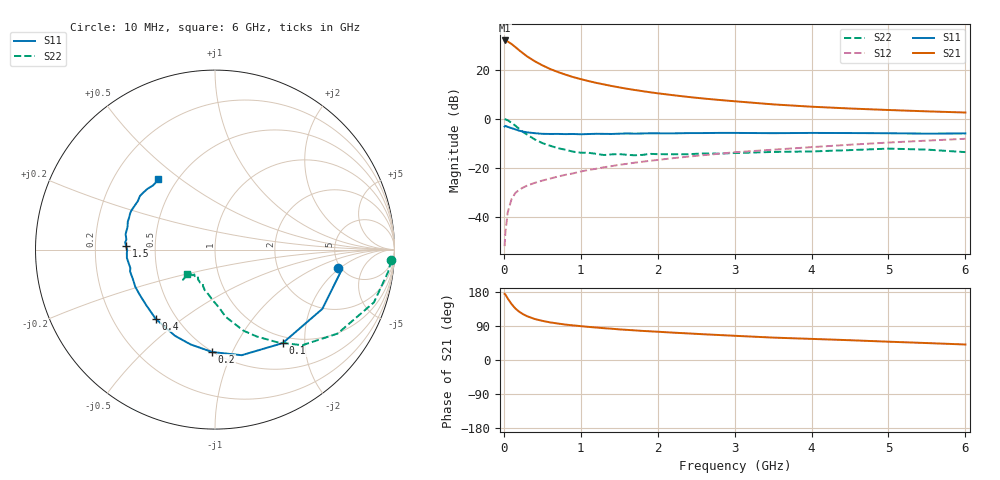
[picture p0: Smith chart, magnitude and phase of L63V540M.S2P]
!  INFINEON TECHNOLOGIES Small Signal Semiconductors
! BFR380L3 , Si-NPN RF-Transistor in TSLP-3-1
!  Vce=3.5 V,  Ic=40 mA
! Common Emitter S-Parameters:  07. March 2005
#  GHz  S  MA  R  50
! f  S11  S21  S12  S22
! GHz  Mag  Ang  Mag  Ang  Mag  Ang  Mag  Ang
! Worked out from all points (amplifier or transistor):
!   36 points, 10 MHz to 6 GHz, reference 50 ohm
!   highest |S21| = 32.0 dB at 10 MHz (marker M1)
!   |S21| within 3 dB of that: start of sweep to 161.4 MHz
!   unconditionally stable (mu >= 1): 1.685 GHz to 4.787 GHz
!   at 250 MHz: K = 0.44, MSG = 27.4 dB, |S12| = -28.1 dB
!   at 1.4 GHz: K = 0.98, MSG = 16.4 dB, |S12| = -19.4 dB
!   at 6 GHz: K = 0.98, MSG = 5.4 dB, |S12| = -8.2 dB
!   S11 on the Smith chart (normalised r, x): 10 MHz: 4.75, -1.84; 100 MHz: 0.89, -1.58; 200 MHz: 0.50, -0.84; 400 MHz: 0.39, -0.40; 1.5 GHz: 0.34, +0.02; 6 GHz: 0.40, +0.42
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0.01  0.692 -8.4  39.74 174.5  0.0025 81.1  0.9842 -3.5
0.02  0.7147 -9.1  39.47 172.9  0.0047 83.4  0.9719 -7.5
0.05  0.6832 -28.9  37.89 162.4  0.0122 77.5  0.9328 -18.4
0.1  0.6432 -54.1  33.68 147.7  0.0228 67.5  0.828 -34.4
0.15  0.6069 -75.8  29.14 135.9  0.0306 62.0  0.7215 -47.6
0.2  0.5709 -91.6  25 127.3  0.0354 57.5  0.6221 -56.1
0.25  0.5456 -104.4  21.69 120.9  0.0393 54.6  0.5355 -64.5
0.3  0.5295 -115.0  18.91 115.7  0.0429 54.1  0.4785 -70.7
0.4  0.5078 -130.7  15.01 108.3  0.049 53.8  0.3797 -80.9
0.5  0.4924 -141.3  12.35 103.3  0.0546 55.2  0.319 -86.6
0.6  0.4892 -149.3  10.41 99.3  0.0599 56.4  0.2819 -92.7
0.7  0.4901 -154.9  9.047 96.3  0.0659 58.0  0.2518 -98.5
0.9  0.4886 -165.6  7.11 91.3  0.0766 60.4  0.213 -108.4
1.1  0.4877 -171.5  5.888 87.4  0.09 62.3  0.2022 -114.1
1.5  0.4954 177.8  4.375 80.8  0.1148 64.6  0.19 -124.1
1.8  0.5007 171.9  3.671 76.8  0.1324 64.9  0.1827 -129.5
2.2  0.5034 165.4  3.03 72.2  0.1568 65.3  0.1882 -132.5
2.8  0.5143 156.5  2.421 65.9  0.1932 65.3  0.1938 -139.0
3.5  0.5079 147.9  1.967 59.1  0.2335 63.5  0.2102 -137.9
4.5  0.5107 141.7  1.62 52.2  0.2951 61.8  0.2289 -137.3
5.5  0.4968 133.8  1.417 44.7  0.3578 58.2  0.2343 -136.8
6  0.5022 128.9  1.341 40.9  0.3903 56.1  0.2083 -138.7
